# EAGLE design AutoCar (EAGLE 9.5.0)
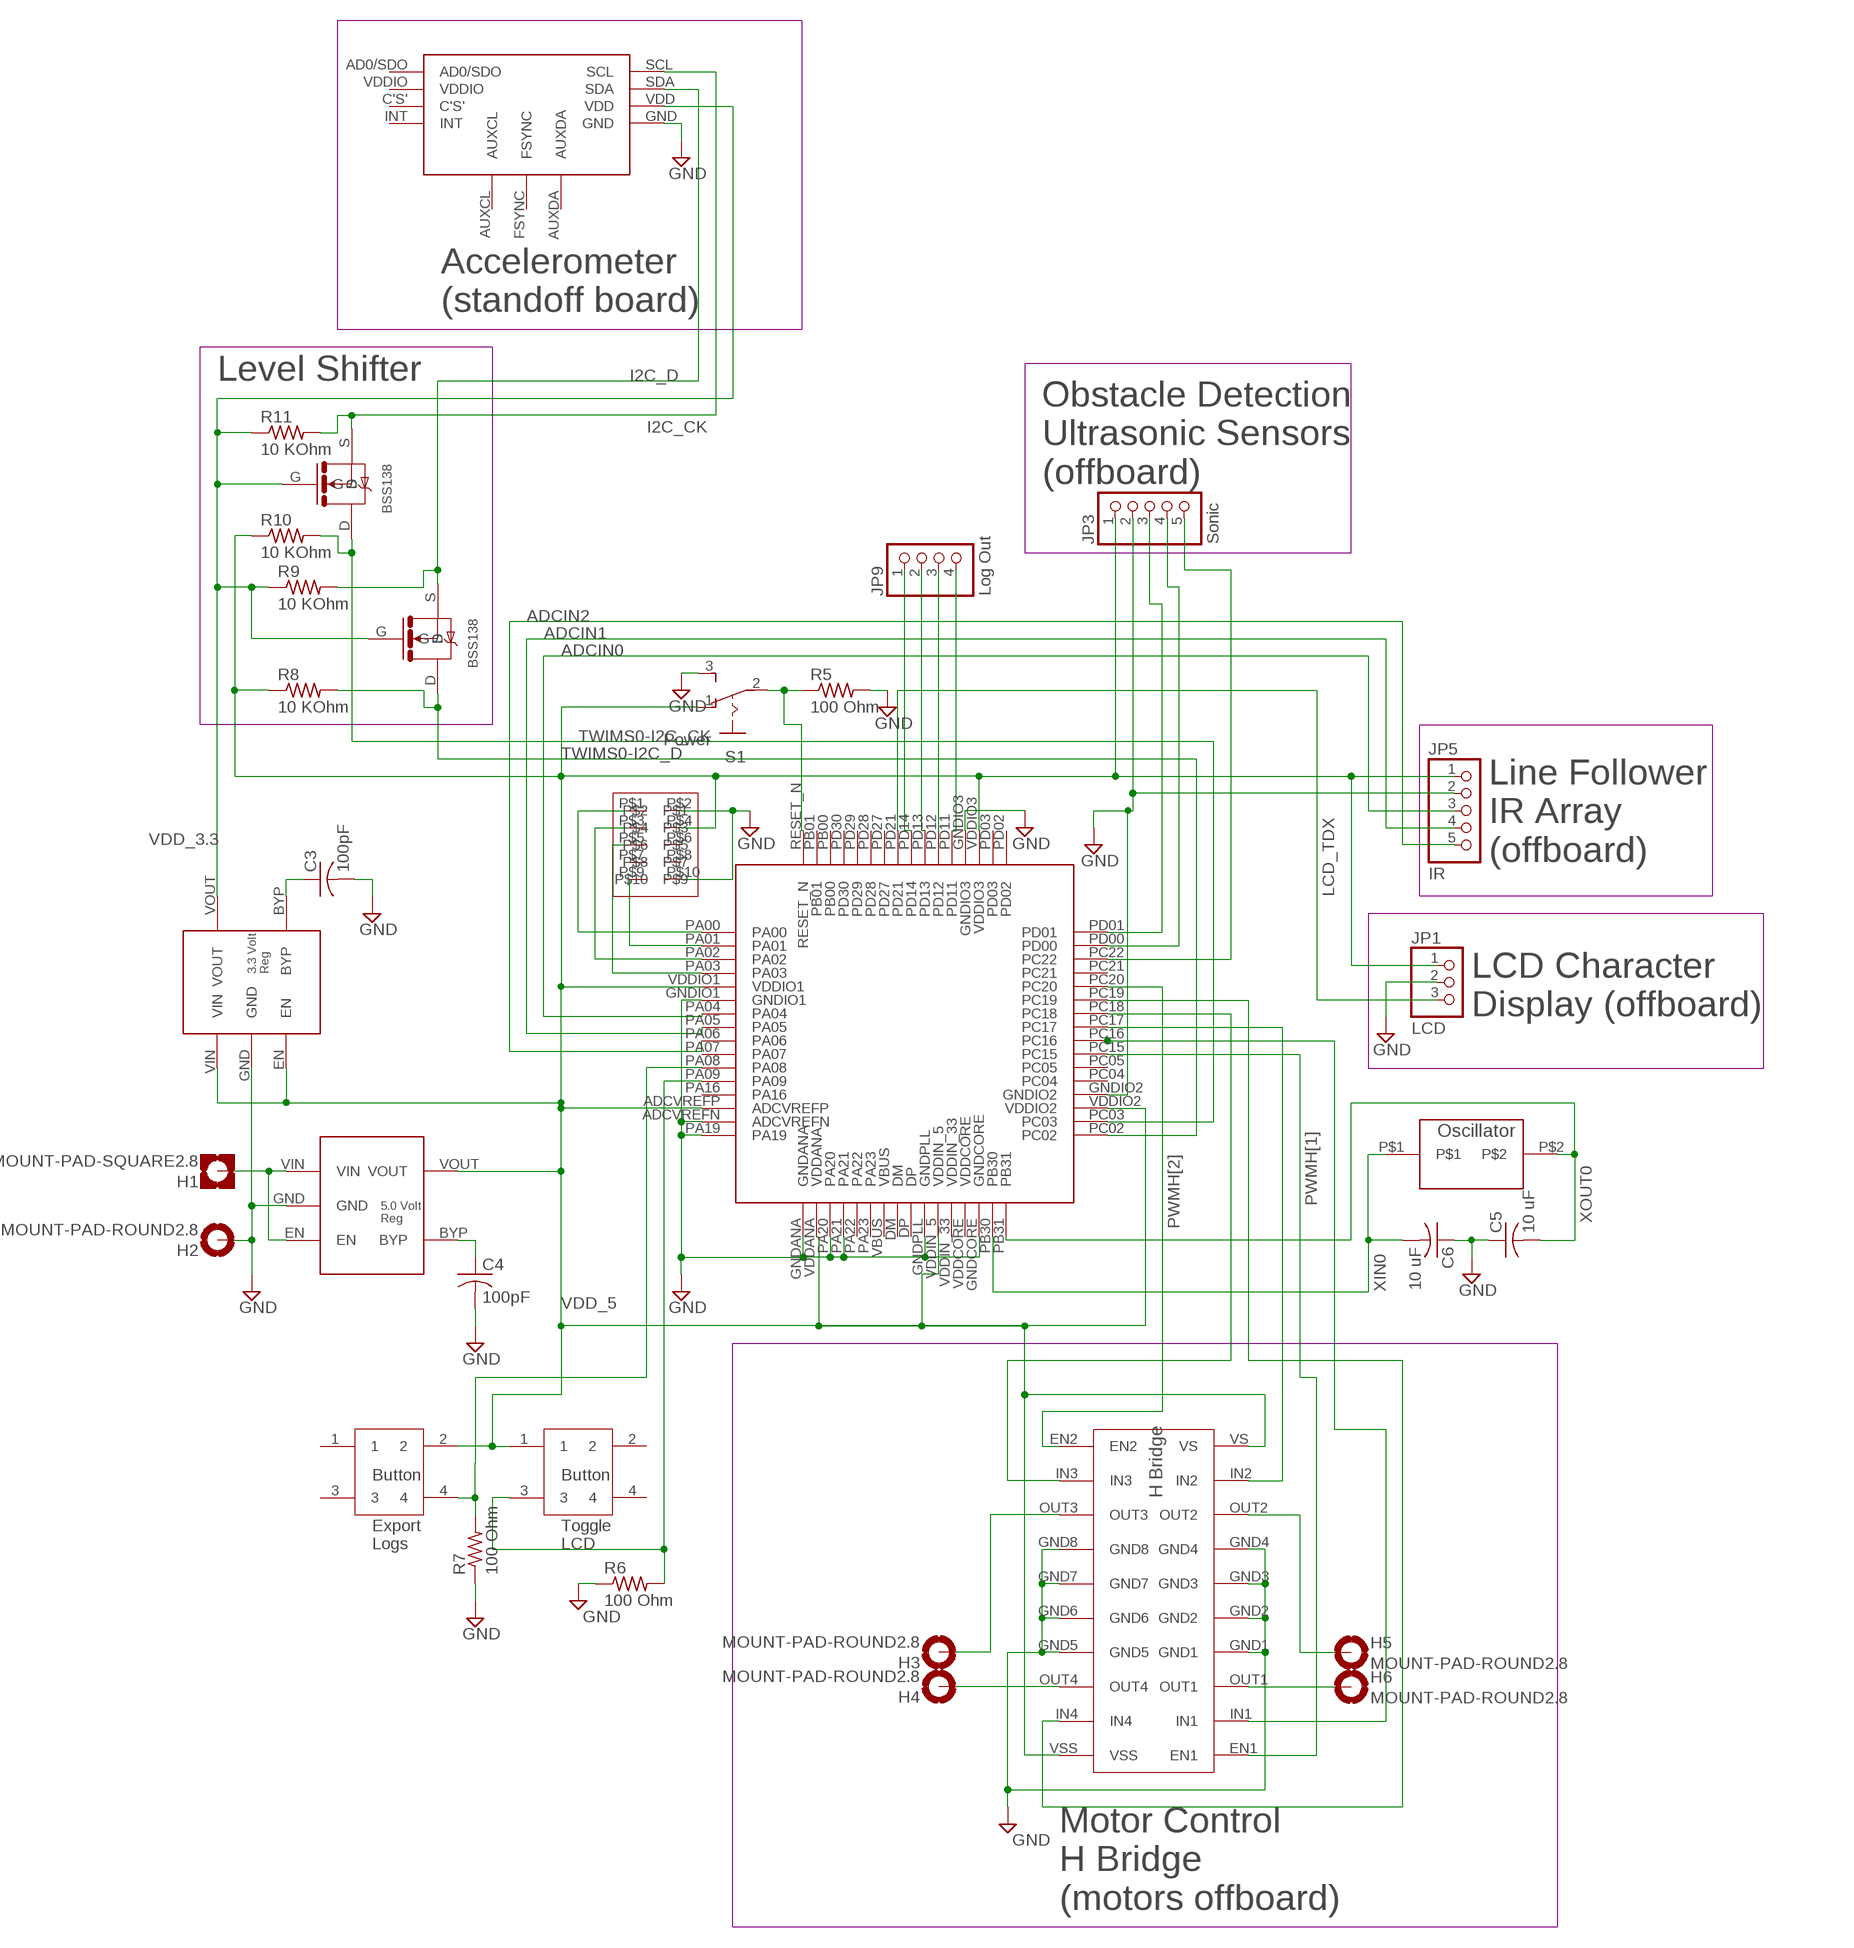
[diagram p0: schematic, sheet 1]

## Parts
C3  100pF  C-USC0805  [C0805]
C4  100pF  C-USC0805  [C0805]
C5  10 uF  C-USC0805  [C0805]
C6  10 uF  C-USC0805  [C0805]
H1  MOUNT-PAD-SQUARE2.8  [2,8-PAD-SQUARE]
H2  MOUNT-PAD-ROUND2.8  [2,8-PAD]
H3  MOUNT-PAD-ROUND2.8  [2,8-PAD]
H4  MOUNT-PAD-ROUND2.8  [2,8-PAD]
H5  MOUNT-PAD-ROUND2.8  [2,8-PAD]
H6  MOUNT-PAD-ROUND2.8  [2,8-PAD]
JP1  LCD  PINHD-1X3  [1X03]
JP3  Sonic  PINHD-1X5  [1X05]
JP5  IR  PINHD-1X5  [1X05]
JP9  Log Out  PINHD-1X4  [1X04]
R5  100 Ohm  R-US_M0805  [M0805]
R6  100 Ohm  R-US_M0805  [M0805]
R7  100 Ohm  R-US_M0805  [M0805]
R8  10 KOhm  R-US_M0805  [M0805]
R9  10 KOhm  R-US_M0805  [M0805]
R10  10 KOhm  R-US_M0805  [M0805]
R11  10 KOhm  R-US_M0805  [M0805]
S1  Power  255SB  [255SB]
U$1  AT32UC3C2512C-A2UT  [TQFP-64]
U$2  GRPB052VWQP-RC  [VWQS5X2]
U$7  AP2210K-5.0TRG1  [SC-74A]
U$8  SEN-13762  [MPU-9250]
U$10  AP2210K-3.3TRG1  [SC-74A]
U$12  L293DD  [SOIC20]
U$14  LFXTAL003210BULK  [HC-49/US]
U$17  PTS645SM43SMTR92LFS  [SM43SMTR92LFS]
U$18  PTS645SM43SMTR92LFS  [SM43SMTR92LFS]
U$19  BSS138  [SOT23]
U$20  BSS138  [SOT23]

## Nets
ADCIN0: JP5.3 U$1.PA04
ADCIN1: JP5.4 U$1.PA05
ADCIN2: JP5.5 U$1.PA06
ECHO_L: JP3.5 U$1.PC22
ECHO_R: JP3.4 U$1.PD00
GND: C3.2 C4.2 C5.1 C6.1 H2.B2,8(MOUNT) JP1.2 JP3.2 JP5.2 R5.2 R6.1 R7.1 S1.3(S) U$1.ADCVREFN U$1.GNDANA U$1.GNDCORE U$1.GNDIO1 U$1.GNDIO2 U$1.GNDIO3 U$1.GNDPLL U$1.PA19 U$1.PA20 U$1.PA21 U$2.P$2 U$2.P$10 U$7.GND U$8.GND U$10.GND U$12.GND1 U$12.GND2 U$12.GND3 U$12.GND4 U$12.GND5 U$12.GND6 U$12.GND7 U$12.GND8
I2C_CK: R11.2 U$8.SCL U$19.S
I2C_D: R9.2 U$8.SDA U$20.S
LCD_TDX: JP1.3 U$1.PD21
N$1: H1.B2,8(MOUNT) U$7.EN U$7.VIN
N$2: H3.B2,8(MOUNT) U$12.OUT3
N$4: H4.B2,8(MOUNT) U$12.OUT4
N$5: H5.B2,8(MOUNT) U$12.OUT2
N$6: H6.B2,8(MOUNT) U$12.OUT1
N$7: JP9.4 U$1.PD11
N$9: JP9.3 U$1.PD12
N$10: R5.1 S1.2(P) U$1.RESET_N
N$11: R6.2 U$1.PA09 U$18.3
N$18: U$1.PC16 U$12.IN1
N$21: U$1.PC19 U$12.IN4
N$22: JP9.1 U$1.PD14
N$23: U$1.PC17 U$12.IN2
N$24: JP9.2 U$1.PD13
N$29: C3.1 U$10.BYP
N$30: C4.1 U$7.BYP
N$32: R7.2 U$1.PA08 U$17.4
N$33: U$1.PC18 U$12.IN3
PWMH[1]: U$1.PC15 U$12.EN1
PWMH[2]: U$1.PC20 U$12.EN2
TCK: U$1.PA00 U$2.P$1
TDI: U$1.PA01 U$2.P$9
TDO: U$1.PA02 U$2.P$3
TMS: U$1.PA03 U$2.P$5
TRIG: JP3.3 U$1.PD01
TWIMS0-I2C_CK: R10.2 U$1.PC03 U$19.D
TWIMS0-I2C_D: R8.2 U$1.PC02 U$20.D
VDD_3.3: R9.1 R11.1 U$8.VDD U$10.VOUT U$19.G U$20.G
VDD_5: JP1.1 JP3.1 JP5.1 R8.1 R10.1 S1.1(O) U$1.ADCVREFP U$1.VDDANA U$1.VDDIN_5 U$1.VDDIO1 U$1.VDDIO2 U$1.VDDIO3 U$2.P$4 U$7.VOUT U$10.EN U$10.VIN U$12.VS U$12.VSS U$17.2 U$18.1
XIN0: C6.2 U$1.PB30 U$14.P$1
XOUT0: C5.2 U$1.PB31 U$14.P$2
Unconnected: U$1.DM U$1.DP U$1.PA07 U$1.PA16 U$1.PA22 U$1.PA23 U$1.PB00 U$1.PB01 U$1.PC04 U$1.PC05 U$1.PC21 U$1.PD02 U$1.PD03 U$1.PD27 U$1.PD28 U$1.PD29 U$1.PD30 U$1.VBUS U$1.VDDCORE U$1.VDDIN_33 U$2.P$6 U$2.P$7 U$2.P$8 U$8.AD0/SDO U$8.AUXCL U$8.AUXDA U$8.C'S' U$8.FSYNC U$8.INT U$8.VDDIO U$17.1 U$17.3 U$18.2 U$18.4

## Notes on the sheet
- Accelerometer
  (standoff board)
- Level Shifter
- Obstacle Detection
  Ultrasonic Sensors
  (offboard)
- Line Follower
  IR Array
  (offboard)
- LCD Character
  Display (offboard)
- Export
  Logs
- Toggle
  LCD
- Motor Control
  H Bridge
  (motors offboard)

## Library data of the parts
C3-C6 = rcl:C-US: CAPACITOR, American symbol; SPICEPREFIX: C
H1 = holes:MOUNT-PAD-SQUARE: MOUNTING PAD, square
H2-H6 = holes:MOUNT-PAD-ROUND: MOUNTING PAD, round
JP1 = pinhead:PINHD-1X3: PIN HEADER
JP3 JP5 = pinhead:PINHD-1X5: PIN HEADER
JP9 = pinhead:PINHD-1X4: PIN HEADER
R5-R11 = rcl:R-US_: RESISTOR, American symbol; SPICEPREFIX: R
S1 = switch:255SB: SLIDING SWITCH Distributor Buerklin, 11G810
U$1 = MILESTONE4LIB_E:AT32UC3C2512C-A2UT
U$2 = MILESTONE4LIB_E:GRPB052VWQP-RC
U$7 = MILESTONE4LIB_E:AP2210K-5.0TRG1
U$8 = miu:SEN-13762
U$10 = MILESTONE4LIB_E:AP2210K-3.3TRG1
U$12 = MILESTONE4LIB_E:L293DD
U$14 = MILESTONE4LIB_E:LFXTAL003210BULK
U$17 U$18 = MILESTONE4LIB_E:PTS645SM43SMTR92LFS
U$19 U$20 = MILESTONE4LIB_E:BSS138

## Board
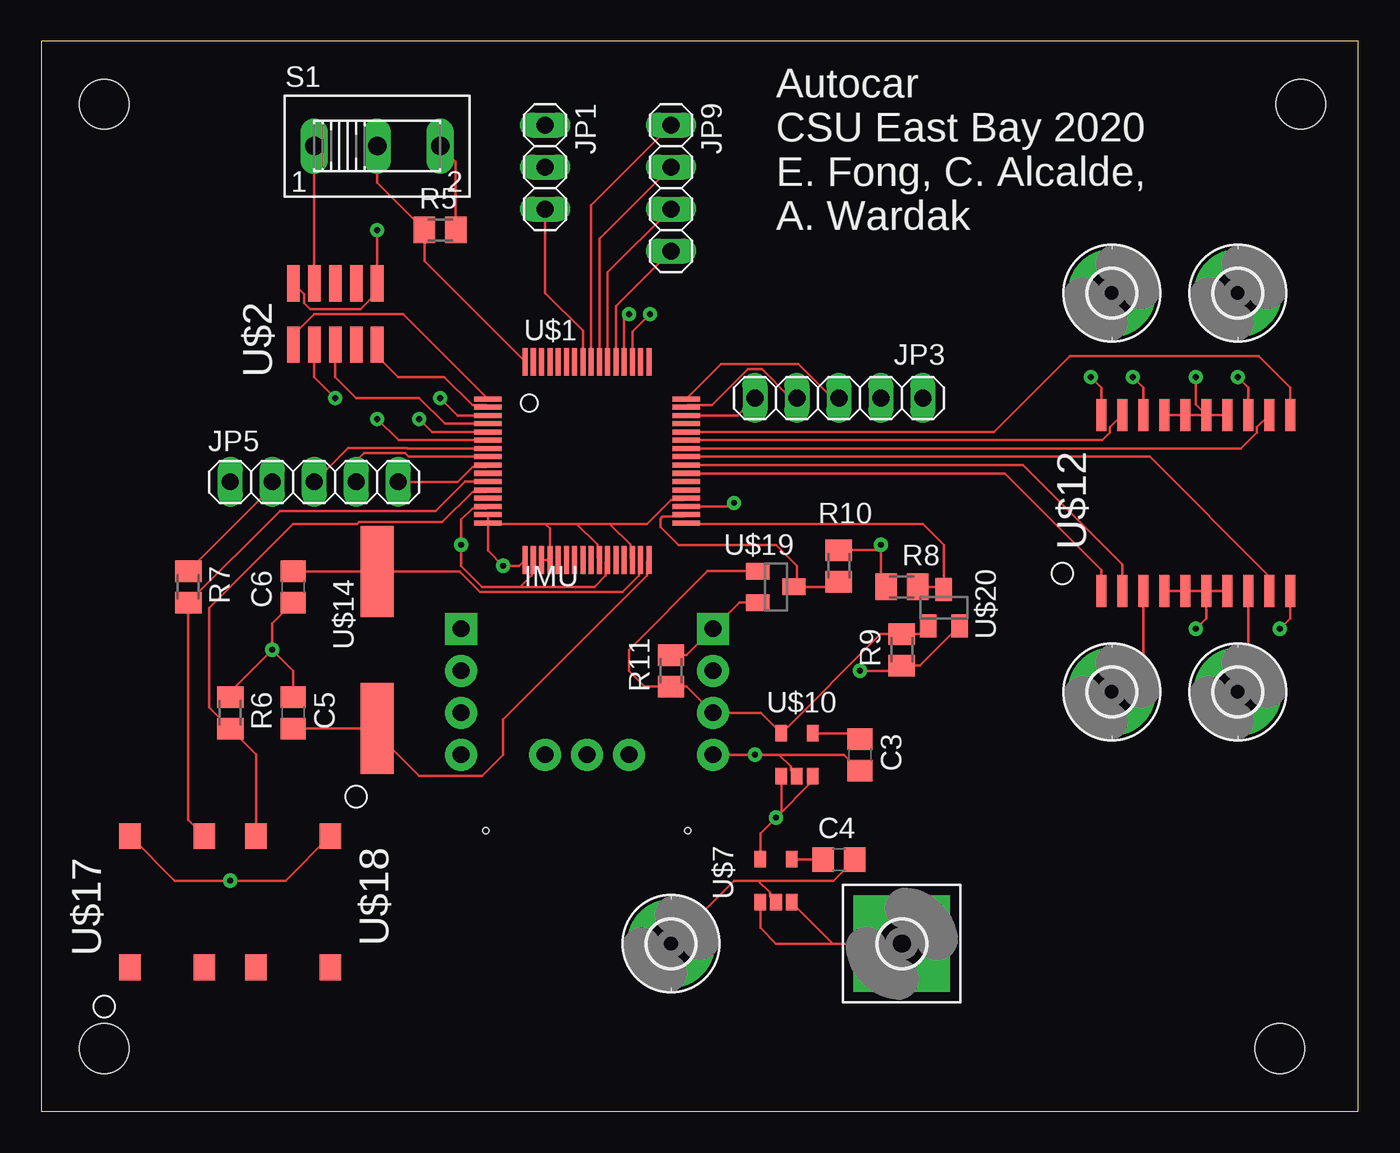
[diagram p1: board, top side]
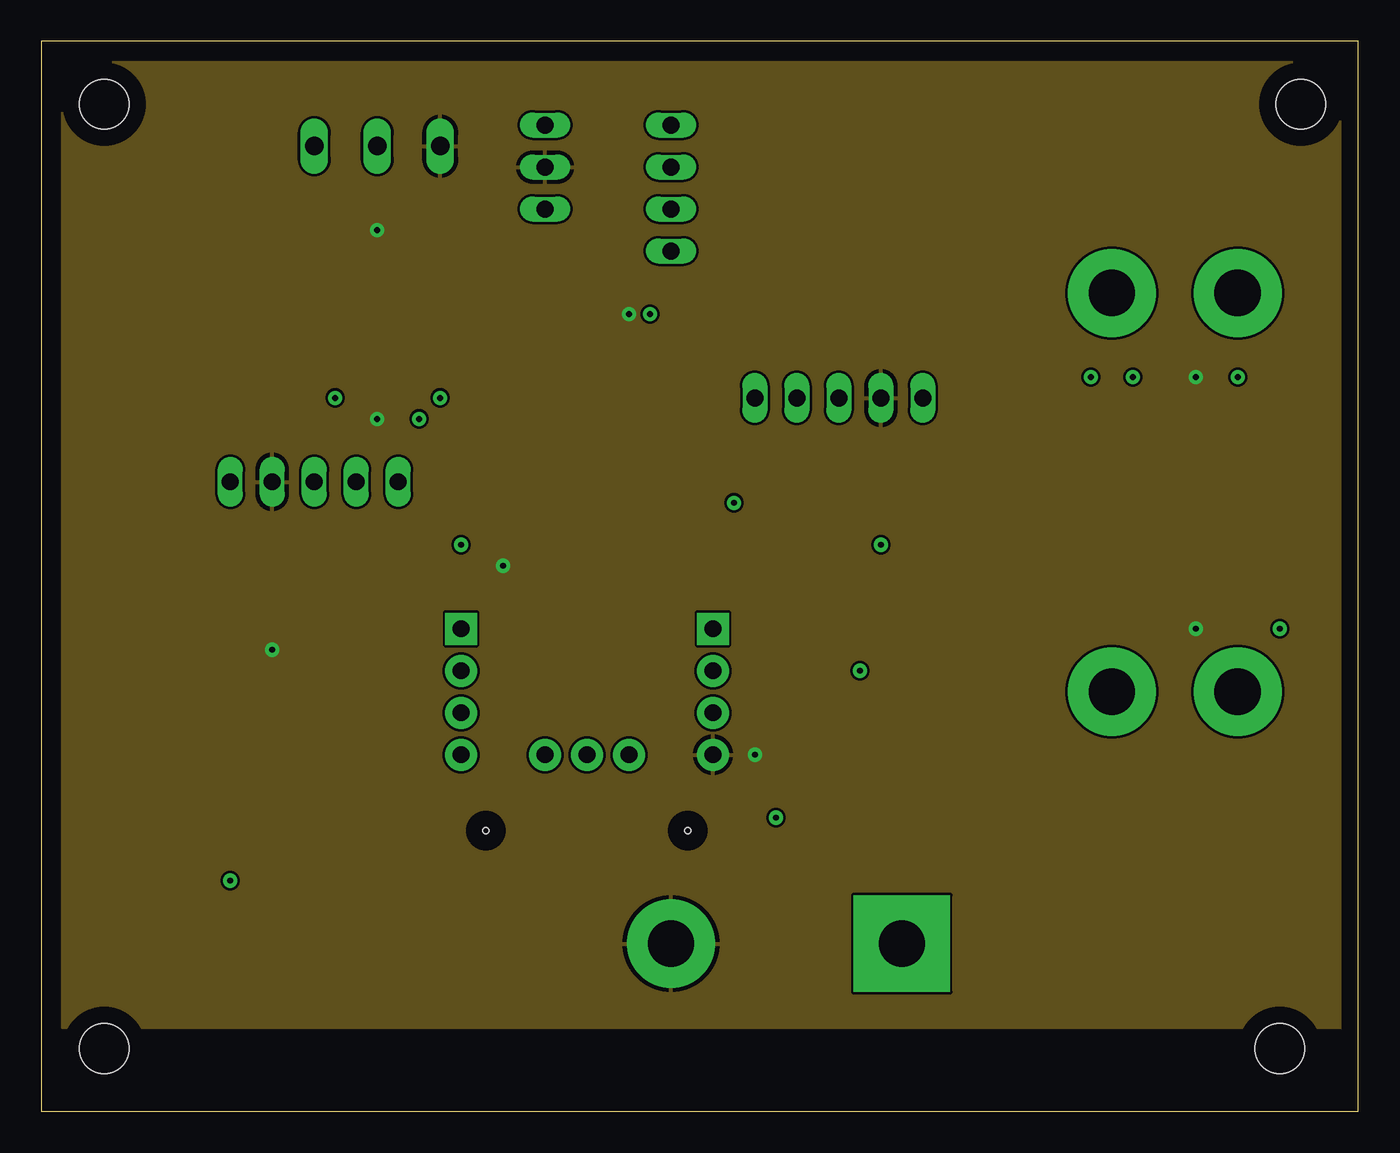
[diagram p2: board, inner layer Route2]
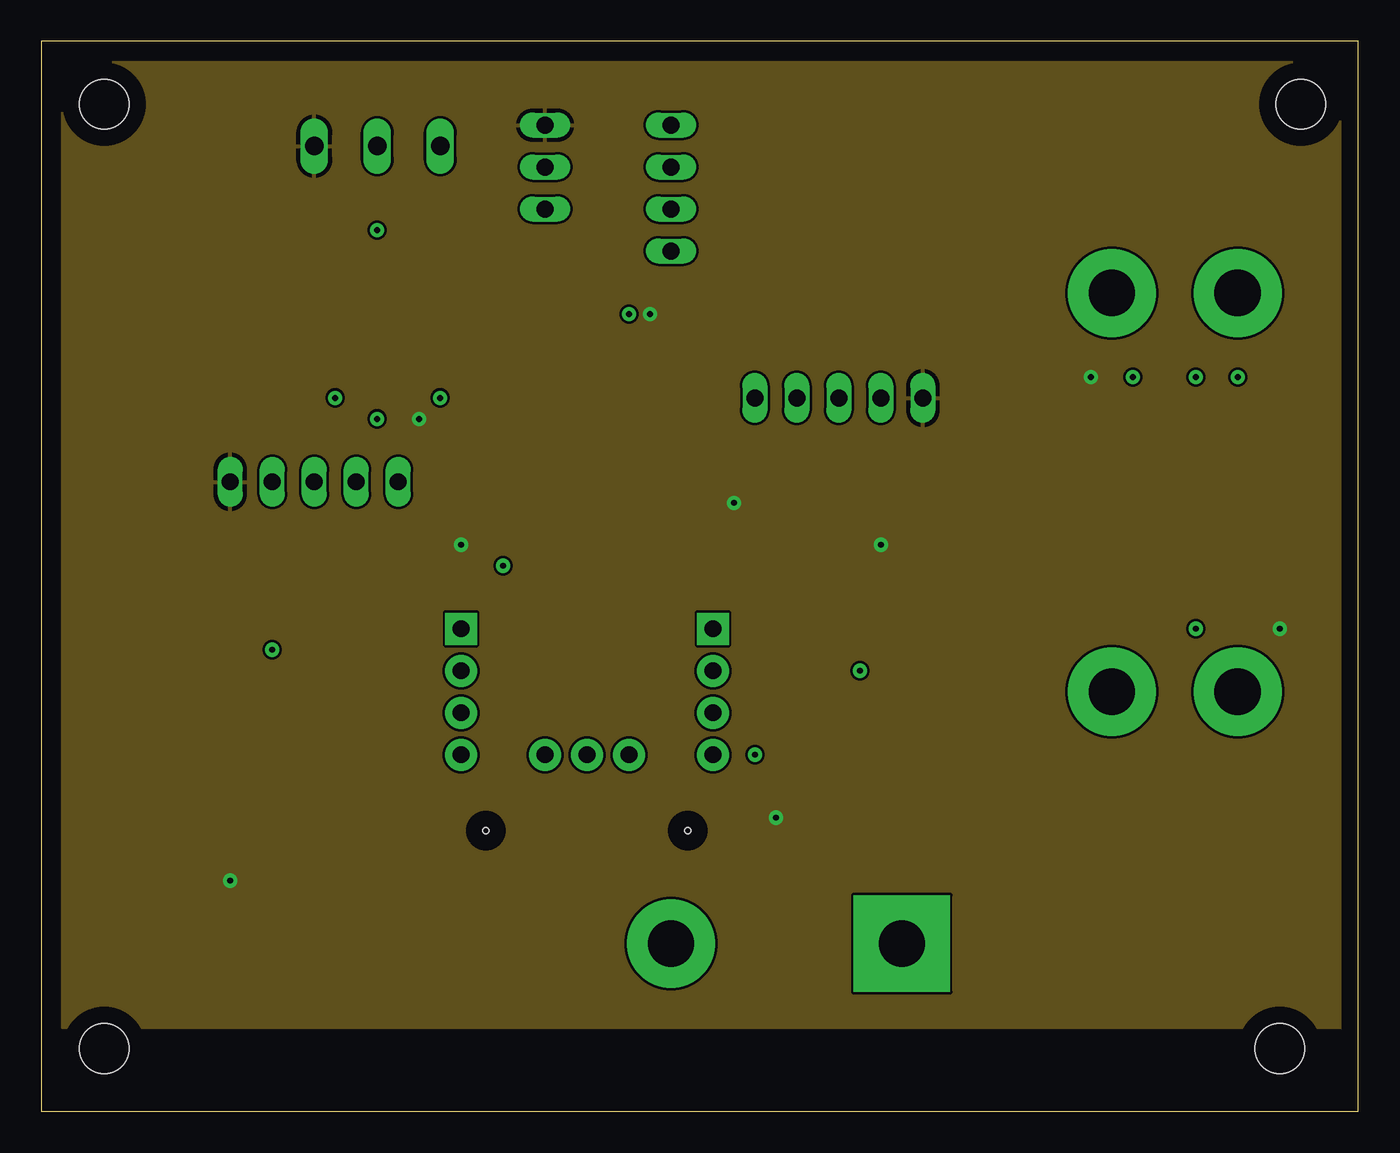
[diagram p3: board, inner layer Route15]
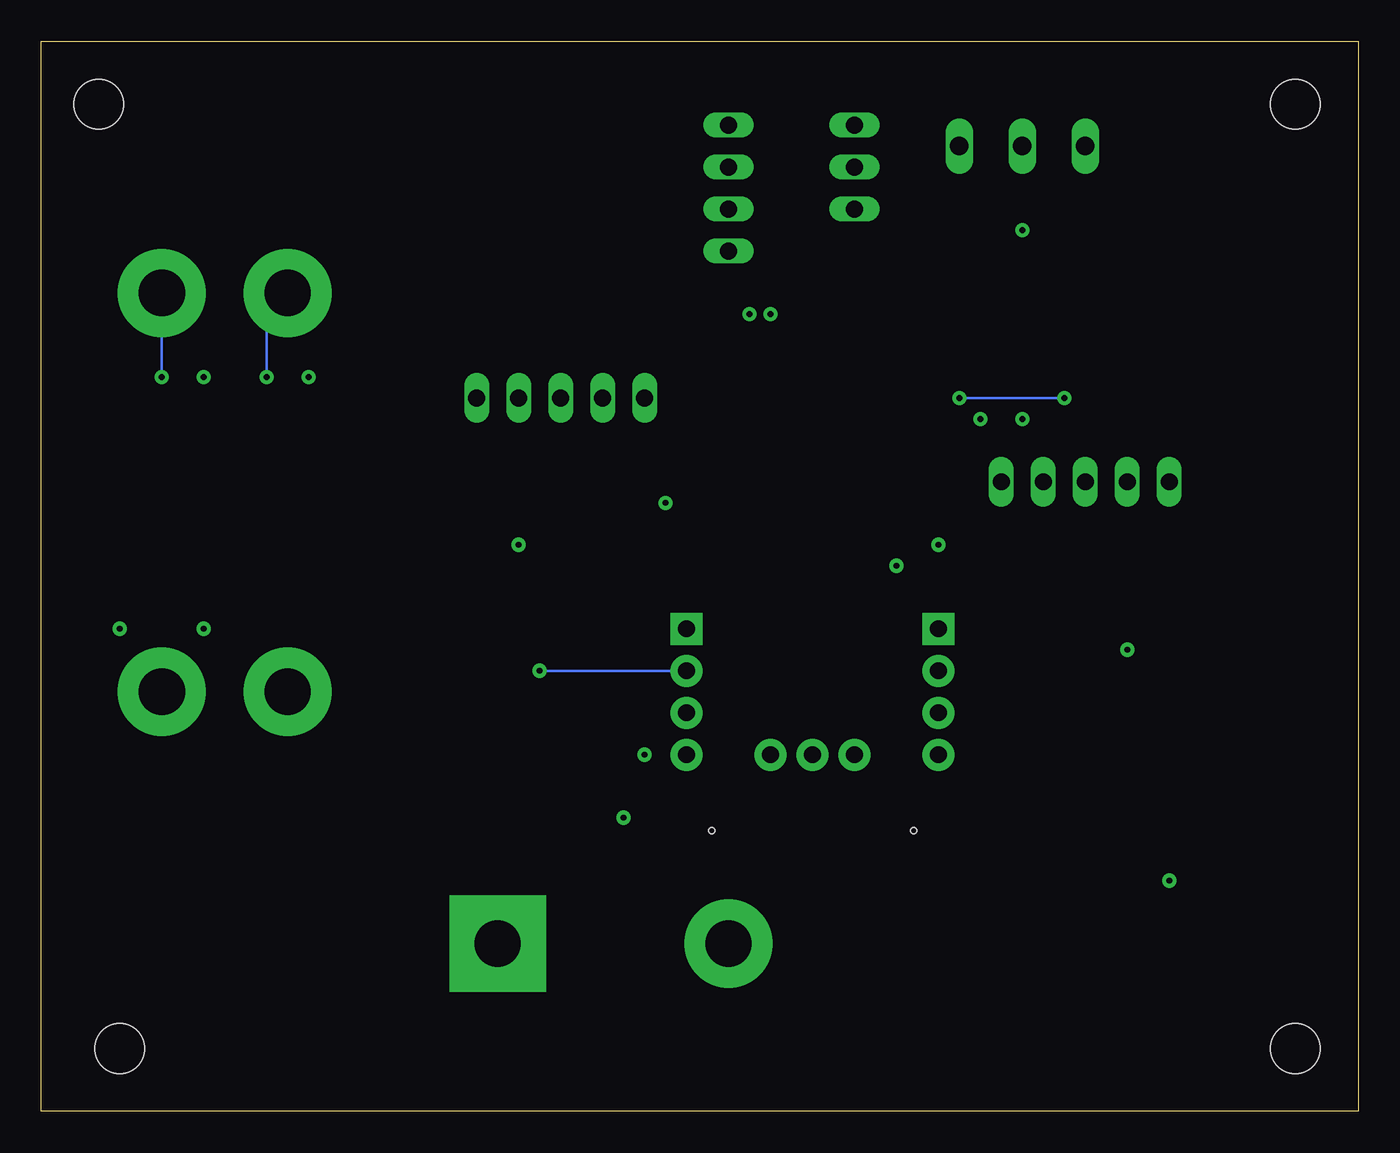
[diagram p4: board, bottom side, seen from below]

Size 79.68 x 64.76 mm. Coordinates in mm from the lower left corner, seen from the top.
Outline: 0,0 79.68,0 79.68,64.76 0,64.76 0,0
Copper layers (1*2*15*16): Top 0.035559375mm / dielectric 62mil / Route2 0.035559375mm / dielectric 62mil / Route15 0.035559375mm / dielectric 62mil / Bottom 0.035559375mm
Design rules "cmpe492-4Layer": minimum track width 6mil, minimum drill 8mil, track to track 6mil, track to pad 6mil, pad to pad 6mil, via to via 6mil, smd to smd 6mil, copper to edge 40mil, drill to drill 20mil, minimum pad ring 10mil, minimum via ring 10mil, stop-mask expansion 4mil, vias tented up to drill 0mil, thermal gap 10mil
Holes 3 mm at 3.81,60.96 76.2,60.96 74.93,3.81 3.81,3.81

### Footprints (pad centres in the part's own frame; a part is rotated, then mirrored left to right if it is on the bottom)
C0805 = smd 1.3 x 1.5: 1 -0.95,0; 2 0.95,0
2,8-PAD-SQUARE = drill 2.8 pad 5.842 square: B2,8 0,0
2,8-PAD = drill 2.8 pad 5.334: B2,8 0,0
1X03 = drill 1.016 long: 1 -2.54,0; 2 0,0; 3 2.54,0
1X05 = drill 1.016 long: 1 -5.08,0; 2 -2.54,0; 3 0,0; 4 2.54,0; 5 5.08,0
1X04 = drill 1.016 long: 1 -3.81,0; 2 -1.27,0; 3 1.27,0; 4 3.81,0
M0805 = smd 1.3 x 1.6: 1 -0.95,0; 2 0.95,0
255SB = drill 1.118 long: 1 -3.81,0; 2 0,0; 3 3.81,0
TQFP-64 = smd 1.676 x 0.305: ADCVREFN -6,-3.25; ADCVREFP -6,-2.75; GNDIO1 -6,1.25; GNDIO2 6,-2.25; PA00 -6,3.75; PA01 -6,3.25; PA02 -6,2.75; PA03 -6,2.25; PA04 -6,0.75; PA05 -6,0.25; PA06 -6,-0.25; PA07 -6,-0.75; PA08 -6,-1.25; PA09 -6,-1.75; PA16 -6,-2.25; PA19 -6,-3.75; PC02 6,-3.75; PC03 6,-3.25; PC04 6,-1.75; PC05 6,-1.25; PC15 6,-0.75; PC16 6,-0.25; PC17 6,0.25; PC18 6,0.75; PC19 6,1.25; PC20 6,1.75; PC21 6,2.25; PC22 6,2.75; PD00 6,3.25; PD01 6,3.75; VDDIO1 -6,1.75; VDDIO2 6,-2.75 | smd 0.305 x 1.676: DM -0.25,-6; DP 0.25,-6; GNDANA -3.75,-6; GNDCORE 2.75,-6; GNDIO3 2.25,6; GNDPLL 0.75,-6; PA20 -2.75,-6; PA21 -2.25,-6; PA22 -1.75,-6; PA23 -1.25,-6; PB00 -2.75,6; PB01 -3.25,6; PB30 3.25,-6; PB31 3.75,-6; PD02 3.75,6; PD03 3.25,6; PD11 1.75,6; PD12 1.25,6; PD13 0.75,6; PD14 0.25,6; PD21 -0.25,6; PD27 -0.75,6; PD28 -1.25,6; PD29 -1.75,6; PD30 -2.25,6; RESET_N -3.75,6; VBUS -0.75,-6; VDDANA -3.25,-6; VDDCORE 2.25,-6; VDDIN_5 1.25,-6; VDDIN_33 1.75,-6; VDDIO3 2.75,6
VWQS5X2 = smd 2.2 x 0.76: P$1 -1.85,2.54; P$2 1.85,2.54; P$3 -1.85,1.27; P$4 1.85,1.27; P$5 -1.85,0; P$6 1.85,0; P$7 -1.85,-1.27; P$8 1.85,-1.27; P$9 -1.85,-2.54; P$10 1.85,-2.54
SC-74A = smd 0.7 x 1: BYP 0.95,1.3; EN 0.95,-1.3; GND 0,-1.3; VIN -0.95,-1.3; VOUT -0.95,1.3
MPU-9250 = drill 1.016 pad 1.93 square: AD0/SDO -7.62,-7.62; SCL -7.62,7.62 | drill 1.016 pad 1.93: AUXCL 0,-2.54; AUXDA 0,2.54; C'S' -2.54,-7.62; FSYNC 0,0; GND 0,7.62; INT 0,-7.62; SDA -5.08,7.62; VDD -2.54,7.62; VDDIO -5.08,-7.62 | hole 0.35: 4.597,-6.121; 4.597,6.096
SOIC20 = smd 0.61 x 1.93: EN1 -5.715,-5.325; EN2 5.715,5.325; GND1 -1.905,-5.325; GND2 -0.635,-5.325; GND3 0.635,-5.325; GND4 1.905,-5.325; GND5 -1.905,5.325; GND6 -0.635,5.325; GND7 0.635,5.325; GND8 1.905,5.325; IN1 -4.445,-5.325; IN2 4.445,-5.325; IN3 4.445,5.325; IN4 -4.445,5.325; OUT1 -3.175,-5.325; OUT2 3.175,-5.325; OUT3 3.175,5.325; OUT4 -3.175,5.325; VS 5.715,-5.325; VSS -5.715,5.325
HC-49/US = smd 5.5 x 2: P$1 -4.75,0; P$2 4.75,0
SM43SMTR92LFS = smd 1.55 x 1.3: 1 -3.975,2.25; 2 3.975,2.25; 3 -3.975,-2.25; 4 3.975,-2.25
SOT23 = smd 1 x 1.4: D 0,1.1; G -0.95,-1.1; S 0.95,-1.1

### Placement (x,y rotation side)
C3  49.53,21.59 270 top
C4  48.26,15.24 0 top
C5  15.24,24.13 270 top
C6  15.24,31.75 90 top
H1  52.07,10.16 0 top
H2  38.1,10.16 0 top
H3  72.39,49.53 0 top
H4  64.77,49.53 0 top
H5  72.39,25.4 0 top
H6  64.77,25.4 0 top
JP1  30.48,57.15 270 top
JP3  48.26,43.18 180 top
JP5  16.51,38.1 0 top
JP9  38.1,55.88 270 top
R5  24.13,53.34 0 top
R6  11.43,24.13 270 top
R7  8.89,31.75 270 top
R8  52.07,31.75 0 top
R9  52.07,27.94 270 top
R10  48.26,33.02 270 top
R11  38.1,26.67 90 top
S1  20.32,58.42 0 top
U$1  33.02,39.37 0 top
U$2  17.78,48.26 90 top
U$7  44.45,13.97 0 top
U$8  33.02,21.59 270 top
U$10  45.72,21.59 0 top
U$12  69.85,36.83 0 top
U$14  20.32,27.94 270 top
U$17  7.62,12.7 90 top
U$18  15.24,12.7 270 top
U$19  44.45,31.75 270 top
U$20  54.61,30.48 0 top

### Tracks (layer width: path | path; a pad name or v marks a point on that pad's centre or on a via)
ADCIN0
  Top 0.152: U$1.PA04 22.16,40.12 22.13,40.16 18.57,40.16 JP5.3
ADCIN1
  Top 0.152: U$1.PA05 22.23,39.62 22,39.85 19.53,39.85 19.05,39.37 JP5.4
ADCIN2
  Top 0.152: U$1.PA06 26.9,39 26.09,39 25.19,38.1 JP5.5
ECHO_L
  Top 0.152: U$1.PC22 42.12,42.12 JP3.5
ECHO_R
  Top 0.152: U$1.PD00 39.14,42.74 40.58,42.74 42.77,44.93 43.59,44.93 45.34,43.18 JP3.4
GND  (via drill 0.35)
  Top 0.152: 30.48,35.56 30.77,35.27 U$1.PA21 U$1.PA20 | U$1.GNDPLL 33.65,33.49 33.65,34.3 32.39,35.56 | 32.39,35.56 30.48,35.56 | U$1.GNDCORE 35.65,33.49 35.65,34.3 34.39,35.56 | 34.39,35.56 32.39,35.56 | 30.48,35.56 27.08,35.56 U$1.PA19 | U$1.PA19 U$1.ADCVREFN | U$12.GND1 U$12.GND2 U$12.GND3 | U$12.GND3 U$12.GND4 | U$12.GND5 U$12.GND6 U$12.GND7 | U$12.GND7 U$12.GND8 | U$10.GND 45.35,20.66 45.35,20.88 44.64,21.59 | 44.64,21.59 v43.18,21.59 U$8.GND | C3.2 48.58,21.59 44.64,21.59 | H2.B2,8 41.91,13.97 43.37,13.97 | U$7.GND 44.08,13.04 44.08,13.27 43.37,13.97 | U$12.GND7 69.85,42.79 v69.85,44.45 | U$12.GND3 70.48,29.84 v69.85,29.21 | C4.2 47.94,13.97 43.37,13.97 | R5.2 25.08,57.47 S1.3 | U$1.GNDIO3 35.27,47.97 v35.56,48.26 | U$1.GNDIO2 38.9,37 38.09,37 36.65,35.56 34.39,35.56 | U$1.PA19 27.02,33.94 v27.94,33.02 28.92,33.02 U$1.GNDANA | U$1.GNDIO1 21.61,40.62 v20.32,41.91 | U$2.P$2 15.9,49.45 15.9,48.91 16.25,48.57 19.31,48.57 20.32,49.58 U$2.P$10 v20.32,53.34 | R7.1 13.97,37.78 JP5.2 | R6.1 11.43,25.4 v13.97,27.94 | C6.1 13.97,29.53 v13.97,27.94 | C5.1 15.24,26.67 v13.97,27.94
  pour Route2: 1.27,63.5 82.55,63.5 82.55,5.08 1.27,5.08
I2C_CK
  Top 0.152: U$19.S 42.23,30.8 U$8.SCL 39.05,27.62 R11.2
I2C_D  (via drill 0.35)
  Top 0.152: U$20.S 53.17,26.99 R9.2 51.75,26.67 v49.53,26.67
  Bottom 0.152: v49.53,26.67 U$8.SDA
LCD_TDX
  Top 0.152: U$1.PD21 32.77,47.24 30.48,49.53 JP1.3
N$1
  Top 0.152: U$7.VIN 43.5,11.11 44.45,10.16 H1.B2,8 47.91,10.16 U$7.EN
N$2  (via drill 0.35)
  Top 0.152: U$12.OUT3 73.03,43.82 v72.39,44.45
  Bottom 0.152: v72.39,44.45 H3.B2,8
N$4  (via drill 0.35)
  Top 0.152: U$12.OUT4 66.67,43.82 v66.04,44.45
  Bottom 0.152: v66.04,44.45 66.04,48.26 H4.B2,8
N$5
  Top 0.152: U$12.OUT2 73.03,26.04 H5.B2,8
N$6
  Top 0.152: U$12.OUT1 66.67,27.3 H6.B2,8
N$7
  Top 0.152: JP9.4 34.77,48.74 U$1.PD11
N$9
  Top 0.152: JP9.3 34.27,50.78 U$1.PD12
N$10
  Top 0.152: U$1.RESET_N 23.18,51.46 R5.1 20.32,56.2 S1.2
N$11
  Top 0.152: U$18.3 12.99,21.62 R6.2 10.16,24.45 10.16,30.48 15.24,35.56 19.12,35.56 19.23,35.67 24.25,35.67 26.09,37.5 26.9,37.5 U$1.PA09
N$18
  Top 0.152: U$1.PC16 59.38,39.12 65.41,33.1 U$12.IN1
N$21
  Top 0.152: U$1.PC19 60.96,40.62 61.54,40.62 64.19,40.62 64.67,41.09 64.67,41.42 U$12.IN4
N$22
  Top 0.152: JP9.1 33.27,54.86 U$1.PD14
N$23
  Top 0.152: U$12.IN2 74.3,32.38 67.06,39.62 U$1.PC17
N$24
  Top 0.152: JP9.2 33.77,52.82 U$1.PD13
N$29
  Top 0.152: U$10.BYP 49.18,22.89 C3.1
N$30
  Top 0.152: U$7.BYP 47.28,15.27 C4.1
N$32
  Top 0.152: U$1.PA08 25.64,38.12 23.86,36.35 14.44,36.35 R7.2 8.89,17.66 U$17.4
N$33
  Top 0.152: U$1.PC18 60.96,40.12 61.61,40.12 72.58,40.12 73.56,41.09 73.56,41.42 U$12.IN3
PWMH[1]
  Top 0.152: U$1.PC15 58.29,38.62 64.14,32.77 U$12.EN1
PWMH[2]
  Top 0.152: U$12.EN2 75.56,43.82 73.66,45.72 62.23,45.72 57.63,41.12 U$1.PC20
TCK
  Top 0.152: U$1.PA00 21.88,48.26 16.51,48.26 15.24,46.99 U$2.P$1
TDI
  Top 0.152: U$1.PA01 26.9,42.74 26.09,42.74 24.38,44.45 21.59,44.45 20.32,45.72 U$2.P$9
TDO  (via drill 0.35)
  Top 0.152: U$1.PA02 25.19,42.12 v24.13,43.18 | v17.78,43.18 16.51,44.45 U$2.P$3
  Bottom 0.152: v24.13,43.18 v17.78,43.18
TMS
  Top 0.152: U$1.PA03 24.42,41.62 22.86,43.18 19.05,43.18 17.78,44.45 U$2.P$5
TRIG
  Top 0.152: JP3.3 47.88,43.18 45.83,45.24 41.14,45.24 U$1.PD01
TWIMS0-I2C_CK
  Top 0.152: U$1.PC03 38.9,36 37.6,36 37.47,35.87 37.47,35.37 38.55,34.29 44.45,34.29 45.72,33.02 45.72,31.92 U$19.D 47.94,31.75 R10.2
TWIMS0-I2C_D
  Top 0.152: U$1.PC02 39.08,35.56 53.34,35.56 54.61,34.29 U$20.D 54.44,31.75 R8.2
VDD_3.3
  Top 0.152: U$19.G 40.32,32.7 35.56,27.94 35.56,26.67 36.51,25.72 R11.1 39.05,25.72 U$8.VDD 43.53,24.13 U$10.VOUT 50.77,28.89 R9.1 53.17,28.89 U$20.G
VDD_5  (via drill 0.35)
  Top 0.152: 44.77,20 U$10.VIN 44.77,18.1 v44.45,17.78 | R10.1 50.8,33.97 v50.8,34.29 50.8,32.07 R8.1 | U$17.2 8.07,13.97 v11.43,13.97 14.79,13.97 U$18.1 | U$7.VOUT 43.5,16.83 v44.45,17.78 | U$12.VSS 64.14,43.82 v63.5,44.45 | U$12.VS 75.56,29.84 v74.93,29.21 | v44.45,17.78 46.67,20 U$10.EN | U$1.ADCVREFP 26.9,36.5 26.09,36.5 25.4,35.81 v25.4,34.29 25.4,33.02 26.67,31.75 28.96,31.75 | U$1.VDDIO3 35.77,47.2 v36.83,48.26 | U$1.VDDIO2 41.7,36.62 v41.91,36.83 | U$1.VDDANA 29.65,33.25 29.65,32.44 28.96,31.75 | U$1.VDDIN_5 34.15,33.25 34.15,32.44 33.46,31.75 28.96,31.75 | U$1.VDDIO1 23.65,41.12 v22.86,41.91 | U$2.P$4 S1.1
  pour Route15: 1.27,63.5 82.55,63.5 82.55,5.08 1.27,5.08
XIN0
  Top 0.152: U$1.PB30 36.15,33.25 36.15,32.44 35.16,31.45 26.54,31.45 25.3,32.69 U$14.P$1 C6.2
XOUT0
  Top 0.152: U$1.PB31 36.65,33.25 36.65,32.44 27.94,23.73 27.94,21.59 26.67,20.32 22.86,20.32 20.32,22.86 U$14.P$2 C5.2

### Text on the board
tNames: Autocar / CSU East Bay 2020 / E. Fong, C. Alcalde, / A. Wardak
